FUNCTION "ValvesLoader" : VOID
TITLE =Valves loader
VERSION : 0.1


VAR_TEMP
  PF_VACUUM_ON : BOOL ;
END_VAR
BEGIN
NETWORK
TITLE =TOGGEL
//Toggle Pushbutton Loader
      U(    ;
      U     "ManualLd";
      U(    ;
      U     "=1+20-S3";
      BLD   100;
      FP    M     16.1;
      )     ;
      =     #PF_VACUUM_ON;
      U     #PF_VACUUM_ON;
      U(    ;
      O     "DO_Pickup (39)";
      ON    "=1+AE32-K7";
      O     "DO_Home (4)";
      )     ;
      U(    ;
      O     "Valvola 1 aspira";
      O     "Valvola 2 aspira";
      )     ;
      O     ;
      U(    ;
      O     "Selez.ciclo sing.ABB";
      O     "Selez. ciclo automatico";
      )     ;
      U     "DO_Vac_On (13)";
      U     "DO_Pickup (39)";
      UN    "Cambio pacco";
      U     "P.E. su tavola soll.";
      )     ;
      S     "M16.0";
      U(    ;
      U     "ManualLd";
      U(    ;
      U     #PF_VACUUM_ON;
      U(    ;
      O     "DO_Home (4)";
      ON    "=1+AE32-K7";
      O     "DO_Pickup (39)";
      )     ;
      O     "DO_Home (4)";
      )     ;
      U(    ;
      ON    "Valvola 1 aspira";
      ON    "Valvola 2 aspira";
      )     ;
      O     ;
      U(    ;
      O     "Selez.ciclo sing.ABB";
      O     "Selez. ciclo automatico";
      )     ;
      U(    ;
      ON    "DO_Vac_On (13)";
      O     "Cambio pacco";
      )     ;
      )     ;
      R     "M16.0";
      NOP   0;
NETWORK
TITLE =ventosa su sfogliatore in aspirazione (ventosa 1)
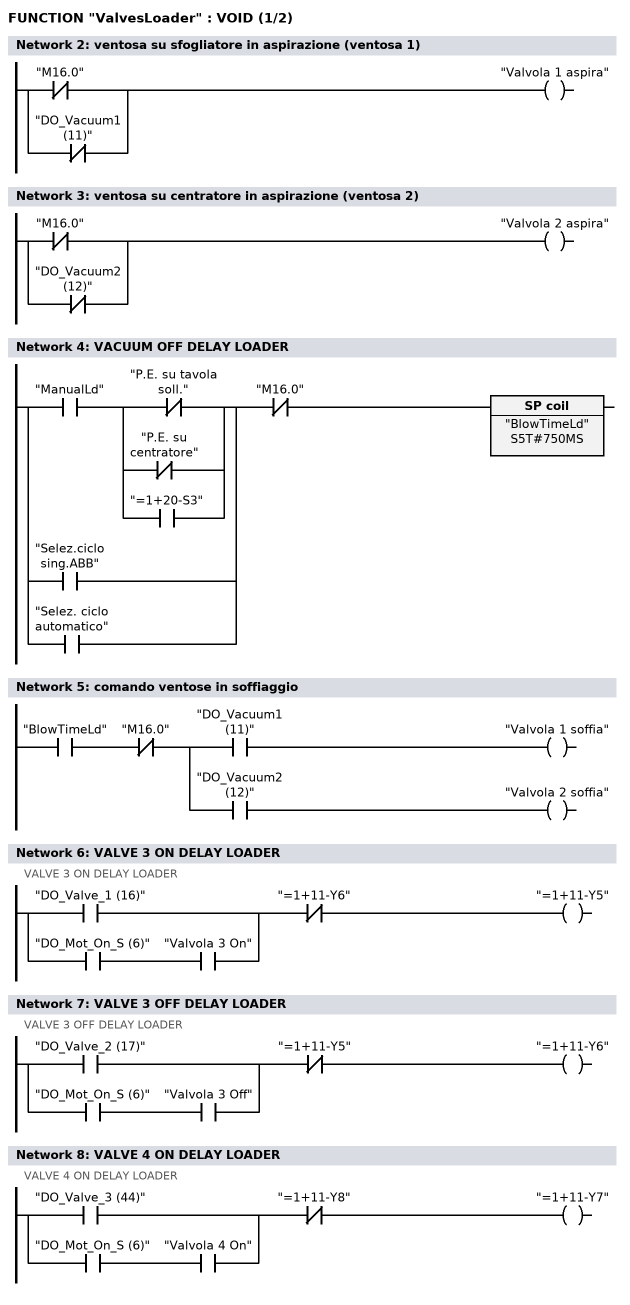
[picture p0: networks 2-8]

      ON    "M16.0";
      ON    "DO_Vacuum1 (11)";
      =     "Valvola 1 aspira";
NETWORK
TITLE =ventosa su centratore in aspirazione (ventosa 2)

      ON    "M16.0";
      ON    "DO_Vacuum2 (12)";
      =     "Valvola 2 aspira";
NETWORK
TITLE =VACUUM OFF DELAY LOADER

      U(    ;
      U     "ManualLd";
      U(    ;
      ON    "P.E. su tavola soll.";
      ON    "P.E. su centratore";
      O     "=1+20-S3";
      )     ;
      O     "Selez.ciclo sing.ABB";
      O     "Selez. ciclo automatico";
      )     ;
      UN    "M16.0";
      L     S5T#750MS;
      SI    "BlowTimeLd";
      NOP   0;
      NOP   0;
      NOP   0;
      NOP   0;
NETWORK
TITLE =comando ventose in soffiaggio

      U     "BlowTimeLd";
      UN    "M16.0";
      =     L      1.0;
      U     L      1.0;
      U     "DO_Vacuum1 (11)";
      =     "Valvola 1 soffia";
      U     L      1.0;
      U     "DO_Vacuum2 (12)";
      =     "Valvola 2 soffia";
NETWORK
TITLE =VALVE 3 ON DELAY LOADER
//VALVE 3 ON DELAY LOADER
      U(    ;
      O     "DO_Valve_1 (16)";
      O     ;
      U     "DO_Mot_On_S (6)";
      U     "Valvola 3 On";
      )     ;
      UN    "=1+11-Y6";
      =     "=1+11-Y5";
NETWORK
TITLE =VALVE 3 OFF DELAY LOADER
//VALVE 3 OFF DELAY LOADER
      U(    ;
      O     "DO_Valve_2 (17)";
      O     ;
      U     "DO_Mot_On_S (6)";
      U     "Valvola 3 Off";
      )     ;
      UN    "=1+11-Y5";
      =     "=1+11-Y6";
NETWORK
TITLE =VALVE 4 ON DELAY LOADER
//VALVE 4 ON DELAY LOADER
      U(    ;
      O     "DO_Valve_3 (44)";
      O     ;
      U     "DO_Mot_On_S (6)";
      U     "Valvola 4 On";
      )     ;
      UN    "=1+11-Y8";
      =     "=1+11-Y7";
NETWORK
TITLE =VALVE 4 OFF DELAY LOADER
//VALVE 4 OFF DELAY LOADER
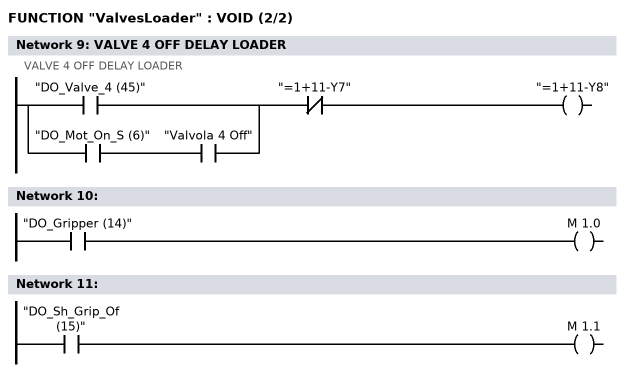
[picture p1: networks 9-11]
      U(    ;
      O     "DO_Valve_4 (45)";
      O     ;
      U     "DO_Mot_On_S (6)";
      U     "Valvola 4 Off";
      )     ;
      UN    "=1+11-Y7";
      =     "=1+11-Y8";
NETWORK
TITLE =

      U     "DO_Gripper (14)";
      =     M      1.0;
NETWORK
TITLE =

      U     "DO_Sh_Grip_Of (15)";
      =     M      1.1;
END_FUNCTION

